(* Logix 5000 AddOnInstructionDefinition export EH_AL1323_8P_CommAOI_Array; software revision 38.00 *)

TYPE EH_CommAOI_Data :
STRUCT
   Device_Comm_Error : BOOL;
   CommSuccess : BOOL;
   CommFailed : BOOL;
   CommTimeOut : BOOL;
   StateDone : BOOL;
   NewState : BOOL;
   OldState : SINT;
   PortSize : SINT;
   DevicePort : SINT;
   MaxState : SINT;
   State : SINT;
   VendorID : INT;
   DeviceID : DINT;
   CyclicData : INT[16];
   AcyclicData : DINT[8];
   ReplayIndex : INT;
   AOI_Diagnostic : DINT;
   ConnectionStatus : DINT;
   OutputData : INT[16];
END_STRUCT
END_TYPE

ADD_ON_INSTRUCTION EH_AL1323_8P_CommAOI_Array   (* revision 1.0, vendor Endress+Hauser *)
// Ethenet/IP Comm AOI for 8 Port IFM AL 1323 with array
// Revision note:
// First Version for the IOLink Communication Block with Array structure in the tag list
VAR_IN_OUT
   Master_InputTag : INT[223]; {required}
   Master_OutputTag : INT[151]; {required}
   DataToSend : INT[10]; {required}
   CommAOIBusy : DINT; {required}
   ActiveComPort : DINT; {required}
   Send_Request : DINT; {required}
   CommError : INT; {required}
   DeviceData : EH_CommAOI_Data; {required}
END_VAR
VAR_INPUT
   iPortSize : INT; {required}
   iDevicePort : INT; {required}
   Master_Input_ConnectionFaulted : BOOL; {required}
END_VAR
VAR
   LocalChannel : DINT; {access None}
   LocalStep : DINT; {access None}
   cChannel : DINT; {access None}
   Port : SINT; {access None}
   count : SINT; {access None}
   PortSize : INT; {access None}
   ChannelData : DINT[15]; {access None}
   TONR_01 : FBD_TIMER; {access None}
   Calc_ConnectionStatus : INT; {access None}
   Calc_VID : INT; {access None}
   Calc_DID : INT; {access None}
   UsedState : INT; {access None}
   DataSendExecuted : BOOL; {access None}
   DataSize : SINT; {access None}
   RW_Input : USINT; {access None}
   RW_Step : USINT; {access None}
   TimerActive : BOOL; {access None}
   ExecuteCounter : DINT; {access None}
END_VAR

ROUTINE Logic   (* structured text *)
   // =======================================================================
   // Endress+Hauser Digital Solutions
   // ©Copyright (2024) All Rights Reserved
   // =======================================================================
   // Name:                EH_AL1323_8P_CommAOI_Array
   // Version:             1.0
   // Datum:               11.2025
   // Library:             01.01.00
   // Engineering:         Studio5000 V38.00.00
   // Author:              EH
   // =======================================================================
   
   
   //Create the Port Config 8P
   	if iDevicePort > 0 and iDevicePort<9 then
   	DeviceData.DevicePort := iDevicePort;
   	else
   	DeviceData.DevicePort := 0;
   	end_if;
   
   	DeviceData.PortSize := iPortSize;
   	DeviceData.Device_Comm_Error := Master_Input_ConnectionFaulted;
   
   
   
   	case DeviceData.PortSize of
   
   		0:
   			PortSize:= 1;
   		1:
   			PortSize:= 2;
   		2:
   			PortSize:= 4;
   		3:
   			PortSize:= 8;
   		4:
   			PortSize:= 16; //16 Int = 32Byte
   
   			DeviceData.AOI_Diagnostic.0 := 0;
   
   		else
   
   			DeviceData.AOI_Diagnostic.0 := 1;
   
   	end_case;
   
   if DeviceData.DevicePort > 0 and DeviceData.DevicePort < 9 then
   
   	Calc_ConnectionStatus := 23+((DeviceData.DevicePort-1)*9);	// Startvalue  23 + Protnumber x Datalength Byte
   	Calc_VID := 24+((DeviceData.DevicePort-1)*9);			// Startvalue  24 + Protnumber x Datalength Byte
   	Calc_DID := 25+((DeviceData.DevicePort-1)*9);
   
   
   
   	//*********************************
   	//Device Connection Status within the Master
   	//*********************************
   
   	if Master_InputTag[Calc_ConnectionStatus] = 1 or Master_InputTag[Calc_ConnectionStatus] = 129 then
   
   	DeviceData.ConnectionStatus := 1; //Good
   
   	else
   
   	DeviceData.ConnectionStatus := 2; //Bad
   
   	end_if;
   
   	//*********************************
   	//Vendor ID
   	//*********************************
   
   	DeviceData.VendorID		:= Master_InputTag[Calc_VID];
   	DeviceData.VendorID.8	:= Master_InputTag[Calc_VID].8;
   	DeviceData.VendorID.9	:= Master_InputTag[Calc_VID].9;
   	DeviceData.VendorID.10	:= Master_InputTag[Calc_VID].10;
   	DeviceData.VendorID.11	:= Master_InputTag[Calc_VID].11;
   	DeviceData.VendorID.12	:= Master_InputTag[Calc_VID].12;
   	DeviceData.VendorID.13	:= Master_InputTag[Calc_VID].13;
   	DeviceData.VendorID.14	:= Master_InputTag[Calc_VID].14;
   	DeviceData.VendorID.15	:= Master_InputTag[Calc_VID].15;
   
   	//*********************************
   	//Device ID
   	//*********************************
   
   
   	DeviceData.DeviceID.0	:= Master_InputTag[Calc_DID].0;
   	DeviceData.DeviceID.1	:= Master_InputTag[Calc_DID].1;
   	DeviceData.DeviceID.2	:= Master_InputTag[Calc_DID].2;
   	DeviceData.DeviceID.3	:= Master_InputTag[Calc_DID].3;
   	DeviceData.DeviceID.4	:= Master_InputTag[Calc_DID].4;
   	DeviceData.DeviceID.5	:= Master_InputTag[Calc_DID].5;
   	DeviceData.DeviceID.6	:= Master_InputTag[Calc_DID].6;
   	DeviceData.DeviceID.7	:= Master_InputTag[Calc_DID].7;
   	DeviceData.DeviceID.8	:= Master_InputTag[Calc_DID].8;
   	DeviceData.DeviceID.9	:= Master_InputTag[Calc_DID].9;
   	DeviceData.DeviceID.10	:= Master_InputTag[Calc_DID].10;
   	DeviceData.DeviceID.11	:= Master_InputTag[Calc_DID].11;
   	DeviceData.DeviceID.12	:= Master_InputTag[Calc_DID].12;
   	DeviceData.DeviceID.13	:= Master_InputTag[Calc_DID].13;
   	DeviceData.DeviceID.14	:= Master_InputTag[Calc_DID].14;
   	DeviceData.DeviceID.15	:= Master_InputTag[Calc_DID].15;
   	DeviceData.DeviceID.16	:= Master_InputTag[Calc_DID+1].0;
   	DeviceData.DeviceID.17	:= Master_InputTag[Calc_DID+1].1;
   	DeviceData.DeviceID.18	:= Master_InputTag[Calc_DID+1].2;
   	DeviceData.DeviceID.19	:= Master_InputTag[Calc_DID+1].3;
   	DeviceData.DeviceID.20	:= Master_InputTag[Calc_DID+1].4;
   	DeviceData.DeviceID.21	:= Master_InputTag[Calc_DID+1].5;
   	DeviceData.DeviceID.22	:= Master_InputTag[Calc_DID+1].6;
   	DeviceData.DeviceID.23	:= Master_InputTag[Calc_DID+1].7;
   	DeviceData.DeviceID.24	:= Master_InputTag[Calc_DID+1].8;
   	DeviceData.DeviceID.25	:= Master_InputTag[Calc_DID+1].9;
   	DeviceData.DeviceID.26	:= Master_InputTag[Calc_DID+1].10;
   	DeviceData.DeviceID.27	:= Master_InputTag[Calc_DID+1].11;
   	DeviceData.DeviceID.28	:= Master_InputTag[Calc_DID+1].12;
   	DeviceData.DeviceID.29	:= Master_InputTag[Calc_DID+1].13;
   	DeviceData.DeviceID.30	:= Master_InputTag[Calc_DID+1].14;
   	DeviceData.DeviceID.31	:= Master_InputTag[Calc_DID+1].15;
   
   	for count := 0 to (PortSize-1) do
   
   			DeviceData.CyclicData[count] := Master_InputTag[(95+count)+((DeviceData.DevicePort-1)*PortSize)];
   			Master_OutputTag[(23+count)+((DeviceData.DevicePort-1)*PortSize)] := DeviceData.OutputData[count];
   	end_for;
   
   
   
   	count:=0;
   
   	end_if;
   
   
   if CommAOIBusy = 0 then
   
   	DeviceData.OldState := 0;
   	DeviceData.CommSuccess := 0;
   	DeviceData.CommTimeOut := 0;
   	DeviceData.ReplayIndex := 0;
   	DataSendExecuted := 0;
   	DataSendExecuted :=0;
   	ExecuteCounter := 0;
   	//TONR_01.Reset := 1;
   
   
   
   end_if;
   
   
   
   	IF Send_Request > 0 and CommAOIBusy = 0 then
   
   		CommAOIBusy := 1;
   
   		for cChannel := 0 to 8 do
   
   			if Send_Request.[cChannel] then
   
   			ActiveComPort := cChannel;
   
   
   			exit;
   
   			end_if;
   
   		end_for;
   
   	end_if;
   
   	if CommAOIBusy = 1
   		and DeviceData.DevicePort = ActiveComPort
   		and DeviceData.StateDone
   		and DeviceData.State > 0
   		and not DataSendExecuted then
   
   		ExecuteCounter := ExecuteCounter +1;
   
   		Master_OutputTag[5].7 := 0;
   		DeviceData.CommSuccess := 0;
   		DeviceData.CommTimeOut := 0;
   
   
   
   		Master_OutputTag[2] := DataToSend[2];		//iDevice_Port;
   		Master_OutputTag[3] := DataToSend[3];		//CMD_Index;
   		Master_OutputTag[4] := DataToSend[4];		//CMD_Subindex;
   		Master_OutputTag[5].0 := DataToSend[5].0;	//CMD_Rd;
   		Master_OutputTag[5].1 := DataToSend[5].1;	//CMD_Wr;
   		Master_OutputTag[5].8 := DataToSend[5].8;	//CMD_ByteLength.0;  // Bits für die Länge
   		Master_OutputTag[5].9 := DataToSend[5].9;	//CMD_ByteLength.1;
   		Master_OutputTag[5].10 := DataToSend[5].10;	//CMD_ByteLength.2;
   		Master_OutputTag[5].11 := DataToSend[5].11;	//CMD_ByteLength.3;
   		Master_OutputTag[5].12 := DataToSend[5].12;	//CMD_ByteLength.4;
   		Master_OutputTag[5].13 := DataToSend[5].13;	//CMD_ByteLength.5;
   		Master_OutputTag[5].14 := DataToSend[5].14;	//CMD_ByteLength.6;
   		Master_OutputTag[5].15 := DataToSend[5].15;	//CMD_ByteLength.7;
   		Master_OutputTag[6] := DataToSend[6];
   		Master_OutputTag[7] := DataToSend[7];
   		Master_OutputTag[8] := DataToSend[8];
   		Master_OutputTag[9] := DataToSend[9];
   
   		Master_OutputTag[5].7 := DataToSend[5].7;	//Trigger
   		/*
   		TONR(TONR_01);
   		TimerActive:= 1;
   		*/
   		DataSendExecuted :=1;
   
   		CommError.0	:= Master_InputTag[5].8;
   		CommError.1	:= Master_InputTag[5].9;
   		CommError.2	:= Master_InputTag[5].10;
   		CommError.3	:= Master_InputTag[5].11;
   		CommError.4	:= Master_InputTag[5].12;
   		CommError.5	:= Master_InputTag[5].13;
   		CommError.6	:= Master_InputTag[5].14;
   		CommError.7	:= Master_InputTag[5].15;
   		DeviceData.NewState := 0;
   
   		if CommError >0 and DataToSend[3] = Master_InputTag[3] then
   
   			DeviceData.AOI_Diagnostic.[DeviceData.State+7] := 1;
   
   		end_if;
   
   end_if;
   
   //*********************
   // Read or write to check if read or write to check for skipped steps
   //*********************
   
   RW_Input.0 := Master_InputTag[5].0;
   RW_Input.1 := Master_InputTag[5].1;
   
   RW_Step.0 := DataToSend[5].0;
   RW_Step.1 := DataToSend[5].1;
   
   
   if Master_InputTag[5].7
   
   	and DeviceData.DevicePort = ActiveComPort
   	and Master_InputTag[3]= Master_OutputTag[3]
   	and DeviceData.State > DeviceData.OldState
   	and RW_Input = RW_Step
   	and DataSendExecuted
   	and DeviceData.State > 0  then
   
       DataSendExecuted :=0;
   	DataSize.0 :=	Master_InputTag[6].0;
   	DataSize.1 :=	Master_InputTag[6].1;
   	DataSize.2 :=	Master_InputTag[6].2;
   	DataSize.3 :=	Master_InputTag[6].3;
   	DataSize.4 :=	Master_InputTag[6].4;
   	DataSize.5 :=	Master_InputTag[6].5;
   	DataSize.6 :=	Master_InputTag[6].6;
   	DataSize.7 :=	Master_InputTag[6].7;
   
   
   	case DataSize of
   
   		0:
   		DeviceData.AcyclicData[0] := 0;
   
   		DeviceData.CommSuccess := 1;
   		DeviceData.StateDone := 0;
   		Master_OutputTag[5].7 := 0;
   
   		DeviceData.ReplayIndex := Master_InputTag[3];
   
   
   		1:
   		DeviceData.AcyclicData[0].0 := Master_InputTag[6].8;
   		DeviceData.AcyclicData[0].1 := Master_InputTag[6].9;
   		DeviceData.AcyclicData[0].2 := Master_InputTag[6].10;
   		DeviceData.AcyclicData[0].3 := Master_InputTag[6].11;
   		DeviceData.AcyclicData[0].4 := Master_InputTag[6].12;
   		DeviceData.AcyclicData[0].5 := Master_InputTag[6].13;
   		DeviceData.AcyclicData[0].6 := Master_InputTag[6].14;
   		DeviceData.AcyclicData[0].7 := Master_InputTag[6].15;
   
   		DeviceData.CommSuccess := 1;
   		DeviceData.StateDone := 0;
   		Master_OutputTag[5].7 := 0;
   
   		DeviceData.ReplayIndex := Master_InputTag[3];
   
   		2:
   		DeviceData.AcyclicData[0].0 := Master_InputTag[7].0;
   		DeviceData.AcyclicData[0].1 := Master_InputTag[7].1;
   		DeviceData.AcyclicData[0].2 := Master_InputTag[7].2;
   		DeviceData.AcyclicData[0].3 := Master_InputTag[7].3;
   		DeviceData.AcyclicData[0].4 := Master_InputTag[7].4;
   		DeviceData.AcyclicData[0].5 := Master_InputTag[7].5;
   		DeviceData.AcyclicData[0].6 := Master_InputTag[7].6;
   		DeviceData.AcyclicData[0].7 := Master_InputTag[7].7;
   		DeviceData.AcyclicData[0].8 := Master_InputTag[6].8;
   		DeviceData.AcyclicData[0].9 := Master_InputTag[6].9;
   		DeviceData.AcyclicData[0].10 := Master_InputTag[6].10;
   		DeviceData.AcyclicData[0].11 := Master_InputTag[6].11;
   		DeviceData.AcyclicData[0].12 := Master_InputTag[6].12;
   		DeviceData.AcyclicData[0].13 := Master_InputTag[6].13;
   		DeviceData.AcyclicData[0].14 := Master_InputTag[6].14;
   		DeviceData.AcyclicData[0].15 := Master_InputTag[6].15;
   
   		DeviceData.CommSuccess := 1;
   		DeviceData.StateDone := 0;
   		Master_OutputTag[5].7 := 0;
   
   		DeviceData.ReplayIndex := Master_InputTag[3];
   
   		4:
   
   		DeviceData.AcyclicData[0].0 := Master_InputTag[8].0;
   		DeviceData.AcyclicData[0].1 := Master_InputTag[8].1;
   		DeviceData.AcyclicData[0].2 := Master_InputTag[8].2;
   		DeviceData.AcyclicData[0].3 := Master_InputTag[8].3;
   		DeviceData.AcyclicData[0].4 := Master_InputTag[8].4;
   		DeviceData.AcyclicData[0].5 := Master_InputTag[8].5;
   		DeviceData.AcyclicData[0].6 := Master_InputTag[8].6;
   		DeviceData.AcyclicData[0].7 := Master_InputTag[8].7;
   		DeviceData.AcyclicData[0].8 := Master_InputTag[7].8;
   		DeviceData.AcyclicData[0].9 := Master_InputTag[7].9;
   		DeviceData.AcyclicData[0].10 := Master_InputTag[7].10;
   		DeviceData.AcyclicData[0].11 := Master_InputTag[7].11;
   		DeviceData.AcyclicData[0].12 := Master_InputTag[7].12;
   		DeviceData.AcyclicData[0].13 := Master_InputTag[7].13;
   		DeviceData.AcyclicData[0].14 := Master_InputTag[7].14;
   		DeviceData.AcyclicData[0].15 := Master_InputTag[7].15;
   	 	DeviceData.AcyclicData[0].16 := Master_InputTag[7].0;
   		DeviceData.AcyclicData[0].17 := Master_InputTag[7].1;
   		DeviceData.AcyclicData[0].18 := Master_InputTag[7].2;
   		DeviceData.AcyclicData[0].19 := Master_InputTag[7].3;
   		DeviceData.AcyclicData[0].20 := Master_InputTag[7].4;
   		DeviceData.AcyclicData[0].21 := Master_InputTag[7].5;
   		DeviceData.AcyclicData[0].22 := Master_InputTag[7].6;
   		DeviceData.AcyclicData[0].23 := Master_InputTag[7].7;
   		DeviceData.AcyclicData[0].24 := Master_InputTag[6].8;
   		DeviceData.AcyclicData[0].25 := Master_InputTag[6].9;
   		DeviceData.AcyclicData[0].26 := Master_InputTag[6].10;
   		DeviceData.AcyclicData[0].27 := Master_InputTag[6].11;
   		DeviceData.AcyclicData[0].28 := Master_InputTag[6].12;
   		DeviceData.AcyclicData[0].29 := Master_InputTag[6].13;
   		DeviceData.AcyclicData[0].30 := Master_InputTag[6].14;
   		DeviceData.AcyclicData[0].31 := Master_InputTag[6].15;
   
   		DeviceData.CommSuccess := 1;
   		DeviceData.StateDone := 0;
   		Master_OutputTag[5].7 := 0;
   
   		DeviceData.ReplayIndex := Master_InputTag[3];
   
   		6:
   
   		DeviceData.AcyclicData[0].0 := Master_InputTag[8].0;
   		DeviceData.AcyclicData[0].1 := Master_InputTag[8].1;
   		DeviceData.AcyclicData[0].2 := Master_InputTag[8].2;
   		DeviceData.AcyclicData[0].3 := Master_InputTag[8].3;
   		DeviceData.AcyclicData[0].4 := Master_InputTag[8].4;
   		DeviceData.AcyclicData[0].5 := Master_InputTag[8].5;
   		DeviceData.AcyclicData[0].6 := Master_InputTag[8].6;
   		DeviceData.AcyclicData[0].7 := Master_InputTag[8].7;
   		DeviceData.AcyclicData[0].8 := Master_InputTag[7].8;
   		DeviceData.AcyclicData[0].9 := Master_InputTag[7].9;
   		DeviceData.AcyclicData[0].10 := Master_InputTag[7].10;
   		DeviceData.AcyclicData[0].11 := Master_InputTag[7].11;
   		DeviceData.AcyclicData[0].12 := Master_InputTag[7].12;
   		DeviceData.AcyclicData[0].13 := Master_InputTag[7].13;
   		DeviceData.AcyclicData[0].14 := Master_InputTag[7].14;
   		DeviceData.AcyclicData[0].15 := Master_InputTag[7].15;
   	 	DeviceData.AcyclicData[0].16 := Master_InputTag[7].0;
   		DeviceData.AcyclicData[0].17 := Master_InputTag[7].1;
   		DeviceData.AcyclicData[0].18 := Master_InputTag[7].2;
   		DeviceData.AcyclicData[0].19 := Master_InputTag[7].3;
   		DeviceData.AcyclicData[0].20 := Master_InputTag[7].4;
   		DeviceData.AcyclicData[0].21 := Master_InputTag[7].5;
   		DeviceData.AcyclicData[0].22 := Master_InputTag[7].6;
   		DeviceData.AcyclicData[0].23 := Master_InputTag[7].7;
   		DeviceData.AcyclicData[0].24 := Master_InputTag[6].8;
   		DeviceData.AcyclicData[0].25 := Master_InputTag[6].9;
   		DeviceData.AcyclicData[0].26 := Master_InputTag[6].10;
   		DeviceData.AcyclicData[0].27 := Master_InputTag[6].11;
   		DeviceData.AcyclicData[0].28 := Master_InputTag[6].12;
   		DeviceData.AcyclicData[0].29 := Master_InputTag[6].13;
   		DeviceData.AcyclicData[0].30 := Master_InputTag[6].14;
   		DeviceData.AcyclicData[0].31 := Master_InputTag[6].15;
   
   		DeviceData.AcyclicData[1].0 := Master_InputTag[9].0;
   		DeviceData.AcyclicData[1].1 := Master_InputTag[9].1;
   		DeviceData.AcyclicData[1].2 := Master_InputTag[9].2;
   		DeviceData.AcyclicData[1].3 := Master_InputTag[9].3;
   		DeviceData.AcyclicData[1].4 := Master_InputTag[9].4;
   		DeviceData.AcyclicData[1].5 := Master_InputTag[9].5;
   		DeviceData.AcyclicData[1].6 := Master_InputTag[9].6;
   		DeviceData.AcyclicData[1].7 := Master_InputTag[9].7;
   		DeviceData.AcyclicData[1].8 :=  Master_InputTag[8].8;
   		DeviceData.AcyclicData[1].9 :=  Master_InputTag[8].9;
   		DeviceData.AcyclicData[1].10 := Master_InputTag[8].10;
   		DeviceData.AcyclicData[1].11 := Master_InputTag[8].11;
   		DeviceData.AcyclicData[1].12 := Master_InputTag[8].12;
   		DeviceData.AcyclicData[1].13 := Master_InputTag[8].13;
   		DeviceData.AcyclicData[1].14 := Master_InputTag[8].14;
   		DeviceData.AcyclicData[1].15 := Master_InputTag[8].15;
   
   		DeviceData.CommSuccess := 1;
   		DeviceData.StateDone := 0;
   		Master_OutputTag[5].7 := 0;
   
   		DeviceData.ReplayIndex := Master_InputTag[3];
   
   		8:
   
   		DeviceData.AcyclicData[0].0 := Master_InputTag[8].0;
   		DeviceData.AcyclicData[0].1 := Master_InputTag[8].1;
   		DeviceData.AcyclicData[0].2 := Master_InputTag[8].2;
   		DeviceData.AcyclicData[0].3 := Master_InputTag[8].3;
   		DeviceData.AcyclicData[0].4 := Master_InputTag[8].4;
   		DeviceData.AcyclicData[0].5 := Master_InputTag[8].5;
   		DeviceData.AcyclicData[0].6 := Master_InputTag[8].6;
   		DeviceData.AcyclicData[0].7 := Master_InputTag[8].7;
   		DeviceData.AcyclicData[0].8 := Master_InputTag[7].8;
   		DeviceData.AcyclicData[0].9 := Master_InputTag[7].9;
   		DeviceData.AcyclicData[0].10 := Master_InputTag[7].10;
   		DeviceData.AcyclicData[0].11 := Master_InputTag[7].11;
   		DeviceData.AcyclicData[0].12 := Master_InputTag[7].12;
   		DeviceData.AcyclicData[0].13 := Master_InputTag[7].13;
   		DeviceData.AcyclicData[0].14 := Master_InputTag[7].14;
   		DeviceData.AcyclicData[0].15 := Master_InputTag[7].15;
   	 	DeviceData.AcyclicData[0].16 := Master_InputTag[7].0;
   		DeviceData.AcyclicData[0].17 := Master_InputTag[7].1;
   		DeviceData.AcyclicData[0].18 := Master_InputTag[7].2;
   		DeviceData.AcyclicData[0].19 := Master_InputTag[7].3;
   		DeviceData.AcyclicData[0].20 := Master_InputTag[7].4;
   		DeviceData.AcyclicData[0].21 := Master_InputTag[7].5;
   		DeviceData.AcyclicData[0].22 := Master_InputTag[7].6;
   		DeviceData.AcyclicData[0].23 := Master_InputTag[7].7;
   		DeviceData.AcyclicData[0].24 := Master_InputTag[6].8;
   		DeviceData.AcyclicData[0].25 := Master_InputTag[6].9;
   		DeviceData.AcyclicData[0].26 := Master_InputTag[6].10;
   		DeviceData.AcyclicData[0].27 := Master_InputTag[6].11;
   		DeviceData.AcyclicData[0].28 := Master_InputTag[6].12;
   		DeviceData.AcyclicData[0].29 := Master_InputTag[6].13;
   		DeviceData.AcyclicData[0].30 := Master_InputTag[6].14;
   		DeviceData.AcyclicData[0].31 := Master_InputTag[6].15;
   
   		DeviceData.AcyclicData[1].0 := Master_InputTag[10].0;
   		DeviceData.AcyclicData[1].1 := Master_InputTag[10].1;
   		DeviceData.AcyclicData[1].2 := Master_InputTag[10].2;
   		DeviceData.AcyclicData[1].3 := Master_InputTag[10].3;
   		DeviceData.AcyclicData[1].4 := Master_InputTag[10].4;
   		DeviceData.AcyclicData[1].5 := Master_InputTag[10].5;
   		DeviceData.AcyclicData[1].6 := Master_InputTag[10].6;
   		DeviceData.AcyclicData[1].7 := Master_InputTag[10].7;
   		DeviceData.AcyclicData[1].8 := Master_InputTag[9].8;
   		DeviceData.AcyclicData[1].9 := Master_InputTag[9].9;
   		DeviceData.AcyclicData[1].10 := Master_InputTag[9].10;
   		DeviceData.AcyclicData[1].11 := Master_InputTag[9].11;
   		DeviceData.AcyclicData[1].12 := Master_InputTag[9].12;
   		DeviceData.AcyclicData[1].13 := Master_InputTag[9].13;
   		DeviceData.AcyclicData[1].14 := Master_InputTag[9].14;
   		DeviceData.AcyclicData[1].15 := Master_InputTag[9].15;
   	 	DeviceData.AcyclicData[1].16 := Master_InputTag[9].0;
   		DeviceData.AcyclicData[1].17 := Master_InputTag[9].1;
   		DeviceData.AcyclicData[1].18 := Master_InputTag[9].2;
   		DeviceData.AcyclicData[1].19 := Master_InputTag[9].3;
   		DeviceData.AcyclicData[1].20 := Master_InputTag[9].4;
   		DeviceData.AcyclicData[1].21 := Master_InputTag[9].5;
   		DeviceData.AcyclicData[1].22 := Master_InputTag[9].6;
   		DeviceData.AcyclicData[1].23 := Master_InputTag[9].7;
   		DeviceData.AcyclicData[1].24 := Master_InputTag[8].8;
   		DeviceData.AcyclicData[1].25 := Master_InputTag[8].9;
   		DeviceData.AcyclicData[1].26 := Master_InputTag[8].10;
   		DeviceData.AcyclicData[1].27 := Master_InputTag[8].11;
   		DeviceData.AcyclicData[1].28 := Master_InputTag[8].12;
   		DeviceData.AcyclicData[1].29 := Master_InputTag[8].13;
   		DeviceData.AcyclicData[1].30 := Master_InputTag[8].14;
   		DeviceData.AcyclicData[1].31 := Master_InputTag[8].15;
   
   		DeviceData.CommSuccess := 1;
   		DeviceData.StateDone := 0;
   		Master_OutputTag[5].7 := 0;
   
   		DeviceData.ReplayIndex := Master_InputTag[3];
   
   	end_case;
   
   
   end_if;
   
END_ROUTINE
END_ADD_ON_INSTRUCTION
